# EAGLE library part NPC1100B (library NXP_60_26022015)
Low Cost Narrow Band Communication Controller The ASIC DLC-3 is a low cost narrow band communication controller MCM (Multi Carrier Modulation) and power line chip. The integrated ARMÒ CortexTM CPU, memory and common interfaces makes it possible to build different systems with a minimum of external components. For communication with DLC-3 the most popular interfaces like Ethernet MII, SPI, several freely configurable serial interfaces and general IO ports for CPU and DSC are included. The ASIC includes all components for a power-line communication while Analog Front End and Power Amplifier are already integrated. With its On-Chip Power-Factor-Correction, Ballast Control and 4 PWM outputs the LCI is a optimal solution for lighting control units. The freely configurable serial interfaces makes it easy to build electronic power meters for smart-metering applications. AAL Eindhoven MK
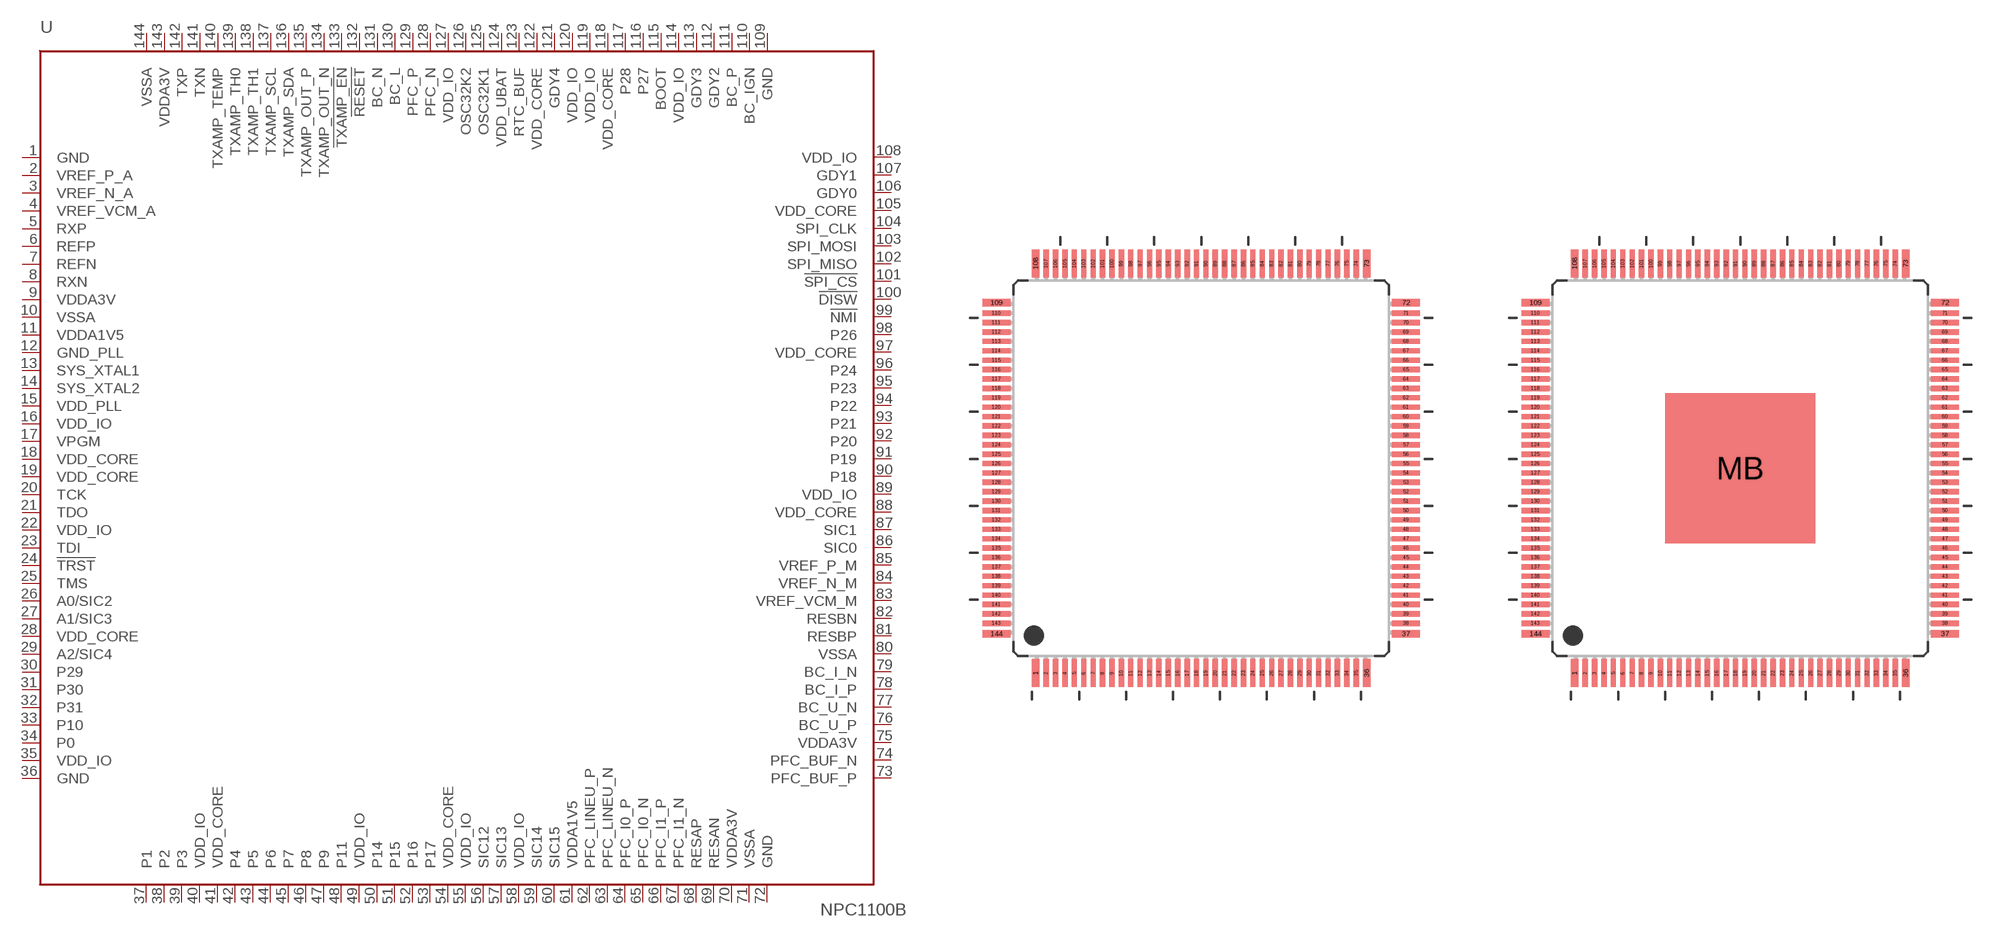
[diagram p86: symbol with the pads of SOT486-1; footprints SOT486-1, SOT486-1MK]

Designator prefix U

## NPC1100B  [SOT486-1]
1  GND
2  VREF_P_A
3  VREF_N_A
4  VREF_VCM_A
5  RXP
6  REFP
7  REFN
8  RXN
9  VDDA3V
10  VSSA
11  VDDA1V5
12  GND_PLL
13  SYS_XTAL1
14  SYS_XTAL2
15  VDD_PLL
16  VDD_IO
17  VPGM
18  VDD_CORE
19  VDD_CORE
20  TCK
21  TDO
22  VDD_IO
23  TDI
24  !TRST!
25  TMS
26  A0/SIC2
27  A1/SIC3
28  VDD_CORE
29  A2/SIC4
30  P29
31  P30
32  P31
33  P10
34  P0
35  VDD_IO
36  GND
37  P1
38  P2
39  P3
40  VDD_IO
41  VDD_CORE
42  P4
43  P5
44  P6
45  P7
46  P8
47  P9
48  P11
49  VDD_IO
50  P14
51  P15
52  P16
53  P17
54  VDD_CORE
55  VDD_IO
56  SIC12
57  SIC13
58  VDD_IO
59  SIC14
60  SIC15
61  VDDA1V5
62  PFC_LINEU_P
63  PFC_LINEU_N
64  PFC_I0_P
65  PFC_I0_N
66  PFC_I1_P
67  PFC_I1_N
68  RESAP
69  RESAN
70  VDDA3V
71  VSSA
72  GND
73  PFC_BUF_P
74  PFC_BUF_N
75  VDDA3V
76  BC_U_P
77  BC_U_N
78  BC_I_P
79  BC_I_N
80  VSSA
81  RESBP
82  RESBN
83  VREF_VCM_M
84  VREF_N_M
85  VREF_P_M
86  SIC0
87  SIC1
88  VDD_CORE
89  VDD_IO
90  P18
91  P19
92  P20
93  P21
94  P22
95  P23
96  P24
97  VDD_CORE
98  P26
99  !NMI!
100  !DISW!
101  !SPI_CS!
102  SPI_MISO
103  SPI_MOSI
104  SPI_CLK
105  VDD_CORE
106  GDY0
107  GDY1
108  VDD_IO
109  GND
110  BC_IGN
111  BC_P
112  GDY2
113  GDY3
114  VDD_IO
115  BOOT
116  P27
117  P28
118  VDD_CORE
119  VDD_IO
120  VDD_IO
121  GDY4
122  VDD_CORE
123  RTC_BUF
124  VDD_UBAT
125  OSC32K1
126  OSC32K2
127  VDD_IO
128  PFC_N
129  PFC_P
130  BC_L
131  BC_N
132  !RESET!
133  !TXAMP_EN!
134  TXAMP_OUT_N
135  TXAMP_OUT_P
136  TXAMP_SDA
137  TXAMP_SCL
138  TXAMP_TH1
139  TXAMP_TH0
140  TXAMP_TEMP
141  TXN
142  TXP
143  VDDA3V
144  VSSA

## NPC1100BCP  [SOT486-1MK]
1  GND
2  VREF_P_A
3  VREF_N_A
4  VREF_VCM_A
5  RXP
6  REFP
7  REFN
8  RXN
9  VDDA3V
10  VSSA
11  VDDA1V5
12  GND_PLL
13  SYS_XTAL1
14  SYS_XTAL2
15  VDD_PLL
16  VDD_IO
17  VPGM
18  VDD_CORE
19  VDD_CORE
20  TCK
21  TDO
22  VDD_IO
23  TDI
24  !TRST!
25  TMS
26  A0/SIC2
27  A1/SIC3
28  VDD_CORE
29  A2/SIC4
30  P29
31  P30
32  P31
33  P10
34  P0
35  VDD_IO
36  GND
37  P1
38  P2
39  P3
40  VDD_IO
41  VDD_CORE
42  P4
43  P5
44  P6
45  P7
46  P8
47  P9
48  P11
49  VDD_IO
50  P14
51  P15
52  P16
53  P17
54  VDD_CORE
55  VDD_IO
56  SIC12
57  SIC13
58  VDD_IO
59  SIC14
60  SIC15
61  VDDA1V5
62  PFC_LINEU_P
63  PFC_LINEU_N
64  PFC_I0_P
65  PFC_I0_N
66  PFC_I1_P
67  PFC_I1_N
68  RESAP
69  RESAN
70  VDDA3V
71  VSSA
72  GND
73  PFC_BUF_P
74  PFC_BUF_N
75  VDDA3V
76  BC_U_P
77  BC_U_N
78  BC_I_P
79  BC_I_N
80  VSSA
81  RESBP
82  RESBN
83  VREF_VCM_M
84  VREF_N_M
85  VREF_P_M
86  SIC0
87  SIC1
88  VDD_CORE
89  VDD_IO
90  P18
91  P19
92  P20
93  P21
94  P22
95  P23
96  P24
97  VDD_CORE
98  P26
99  !NMI!
100  !DISW!
101  !SPI_CS!
102  SPI_MISO
103  SPI_MOSI
104  SPI_CLK
105  VDD_CORE
106  GDY0
107  GDY1
108  VDD_IO
109  GND
110  BC_IGN
111  BC_P
112  GDY2
113  GDY3
114  VDD_IO
115  BOOT
116  P27
117  P28
118  VDD_CORE
119  VDD_IO
120  VDD_IO
121  GDY4
122  VDD_CORE
123  RTC_BUF
124  VDD_UBAT
125  OSC32K1
126  OSC32K2
127  VDD_IO
128  PFC_N
129  PFC_P
130  BC_L
131  BC_N
132  !RESET!
133  !TXAMP_EN!
134  TXAMP_OUT_N
135  TXAMP_OUT_P
136  TXAMP_SDA
137  TXAMP_SCL
138  TXAMP_TH1
139  TXAMP_TH0
140  TXAMP_TEMP
141  TXN
142  TXP
143  VDDA3V
144  VSSA
MB  GND

## Footprint SOT486-1 (pad centres in mm)
SOT486-1 LQFP144: plastic low profile quad flat package; 144 leads; body 20 x 20 x 1.4 mm JEDEC: MS-026 IEC: 136E23
smd 0.4 x 1.5: 1 -8.81,-10.9; 36 8.81,-10.9; 73 8.81,10.9; 108 -8.81,10.9
smd 0.28 x 1.5: 2 -8.25,-10.9; 3 -7.75,-10.9; 4 -7.25,-10.9; 5 -6.75,-10.9; 6 -6.25,-10.9; 7 -5.75,-10.9; 8 -5.25,-10.9; 9 -4.75,-10.9; 10 -4.25,-10.9; 11 -3.75,-10.9; 12 -3.25,-10.9; 13 -2.75,-10.9; 14 -2.25,-10.9; 15 -1.75,-10.9; 16 -1.25,-10.9; 17 -0.75,-10.9; 18 -0.25,-10.9; 19 0.25,-10.9; 20 0.75,-10.9; 21 1.25,-10.9; 22 1.75,-10.9; 23 2.25,-10.9; 24 2.75,-10.9; 25 3.25,-10.9; 26 3.75,-10.9; 27 4.25,-10.9; 28 4.75,-10.9; 29 5.25,-10.9; 30 5.75,-10.9; 31 6.25,-10.9; 32 6.75,-10.9; 33 7.25,-10.9; 34 7.75,-10.9; 35 8.25,-10.9; 74 8.25,10.9; 75 7.75,10.9; 76 7.25,10.9; 77 6.75,10.9; 78 6.25,10.9; 79 5.75,10.9; 80 5.25,10.9; 81 4.75,10.9; 82 4.25,10.9; 83 3.75,10.9; 84 3.25,10.9; 85 2.75,10.9; 86 2.25,10.9; 87 1.75,10.9; 88 1.25,10.9; 89 0.75,10.9; 90 0.25,10.9; 91 -0.25,10.9; 92 -0.75,10.9; 93 -1.25,10.9; 94 -1.75,10.9; 95 -2.25,10.9; 96 -2.75,10.9; 97 -3.25,10.9; 98 -3.75,10.9; 99 -4.25,10.9; 100 -4.75,10.9; 101 -5.25,10.9; 102 -5.75,10.9; 103 -6.25,10.9; 104 -6.75,10.9; 105 -7.25,10.9; 106 -7.75,10.9; 107 -8.25,10.9
smd 1.5 x 0.4: 37 10.9,-8.81; 72 10.9,8.81; 109 -10.9,8.81; 144 -10.9,-8.81
smd 1.5 x 0.28: 38 10.9,-8.25; 39 10.9,-7.75; 40 10.9,-7.25; 41 10.9,-6.75; 42 10.9,-6.25; 43 10.9,-5.75; 44 10.9,-5.25; 45 10.9,-4.75; 46 10.9,-4.25; 47 10.9,-3.75; 48 10.9,-3.25; 49 10.9,-2.75; 50 10.9,-2.25; 51 10.9,-1.75; 52 10.9,-1.25; 53 10.9,-0.75; 54 10.9,-0.25; 55 10.9,0.25; 56 10.9,0.75; 57 10.9,1.25; 58 10.9,1.75; 59 10.9,2.25; 60 10.9,2.75; 61 10.9,3.25; 62 10.9,3.75; 63 10.9,4.25; 64 10.9,4.75; 65 10.9,5.25; 66 10.9,5.75; 67 10.9,6.25; 68 10.9,6.75; 69 10.9,7.25; 70 10.9,7.75; 71 10.9,8.25; 110 -10.9,8.25; 111 -10.9,7.75; 112 -10.9,7.25; 113 -10.9,6.75; 114 -10.9,6.25; 115 -10.9,5.75; 116 -10.9,5.25; 117 -10.9,4.75; 118 -10.9,4.25; 119 -10.9,3.75; 120 -10.9,3.25; 121 -10.9,2.75; 122 -10.9,2.25; 123 -10.9,1.75; 124 -10.9,1.25; 125 -10.9,0.75; 126 -10.9,0.25; 127 -10.9,-0.25; 128 -10.9,-0.75; 129 -10.9,-1.25; 130 -10.9,-1.75; 131 -10.9,-2.25; 132 -10.9,-2.75; 133 -10.9,-3.25; 134 -10.9,-3.75; 135 -10.9,-4.25; 136 -10.9,-4.75; 137 -10.9,-5.25; 138 -10.9,-5.75; 139 -10.9,-6.25; 140 -10.9,-6.75; 141 -10.9,-7.25; 142 -10.9,-7.75; 143 -10.9,-8.25

## Footprint SOT486-1MK (pad centres in mm)
smd 0.4 x 1.5: 1 -8.81,-10.9; 36 8.81,-10.9; 73 8.81,10.9; 108 -8.81,10.9
smd 0.28 x 1.5: 2 -8.25,-10.9; 3 -7.75,-10.9; 4 -7.25,-10.9; 5 -6.75,-10.9; 6 -6.25,-10.9; 7 -5.75,-10.9; 8 -5.25,-10.9; 9 -4.75,-10.9; 10 -4.25,-10.9; 11 -3.75,-10.9; 12 -3.25,-10.9; 13 -2.75,-10.9; 14 -2.25,-10.9; 15 -1.75,-10.9; 16 -1.25,-10.9; 17 -0.75,-10.9; 18 -0.25,-10.9; 19 0.25,-10.9; 20 0.75,-10.9; 21 1.25,-10.9; 22 1.75,-10.9; 23 2.25,-10.9; 24 2.75,-10.9; 25 3.25,-10.9; 26 3.75,-10.9; 27 4.25,-10.9; 28 4.75,-10.9; 29 5.25,-10.9; 30 5.75,-10.9; 31 6.25,-10.9; 32 6.75,-10.9; 33 7.25,-10.9; 34 7.75,-10.9; 35 8.25,-10.9; 74 8.25,10.9; 75 7.75,10.9; 76 7.25,10.9; 77 6.75,10.9; 78 6.25,10.9; 79 5.75,10.9; 80 5.25,10.9; 81 4.75,10.9; 82 4.25,10.9; 83 3.75,10.9; 84 3.25,10.9; 85 2.75,10.9; 86 2.25,10.9; 87 1.75,10.9; 88 1.25,10.9; 89 0.75,10.9; 90 0.25,10.9; 91 -0.25,10.9; 92 -0.75,10.9; 93 -1.25,10.9; 94 -1.75,10.9; 95 -2.25,10.9; 96 -2.75,10.9; 97 -3.25,10.9; 98 -3.75,10.9; 99 -4.25,10.9; 100 -4.75,10.9; 101 -5.25,10.9; 102 -5.75,10.9; 103 -6.25,10.9; 104 -6.75,10.9; 105 -7.25,10.9; 106 -7.75,10.9; 107 -8.25,10.9
smd 1.5 x 0.4: 37 10.9,-8.81; 72 10.9,8.81; 109 -10.9,8.81; 144 -10.9,-8.81
smd 1.5 x 0.28: 38 10.9,-8.25; 39 10.9,-7.75; 40 10.9,-7.25; 41 10.9,-6.75; 42 10.9,-6.25; 43 10.9,-5.75; 44 10.9,-5.25; 45 10.9,-4.75; 46 10.9,-4.25; 47 10.9,-3.75; 48 10.9,-3.25; 49 10.9,-2.75; 50 10.9,-2.25; 51 10.9,-1.75; 52 10.9,-1.25; 53 10.9,-0.75; 54 10.9,-0.25; 55 10.9,0.25; 56 10.9,0.75; 57 10.9,1.25; 58 10.9,1.75; 59 10.9,2.25; 60 10.9,2.75; 61 10.9,3.25; 62 10.9,3.75; 63 10.9,4.25; 64 10.9,4.75; 65 10.9,5.25; 66 10.9,5.75; 67 10.9,6.25; 68 10.9,6.75; 69 10.9,7.25; 70 10.9,7.75; 71 10.9,8.25; 110 -10.9,8.25; 111 -10.9,7.75; 112 -10.9,7.25; 113 -10.9,6.75; 114 -10.9,6.25; 115 -10.9,5.75; 116 -10.9,5.25; 117 -10.9,4.75; 118 -10.9,4.25; 119 -10.9,3.75; 120 -10.9,3.25; 121 -10.9,2.75; 122 -10.9,2.25; 123 -10.9,1.75; 124 -10.9,1.25; 125 -10.9,0.75; 126 -10.9,0.25; 127 -10.9,-0.25; 128 -10.9,-0.75; 129 -10.9,-1.25; 130 -10.9,-1.75; 131 -10.9,-2.25; 132 -10.9,-2.75; 133 -10.9,-3.25; 134 -10.9,-3.75; 135 -10.9,-4.25; 136 -10.9,-4.75; 137 -10.9,-5.25; 138 -10.9,-5.75; 139 -10.9,-6.25; 140 -10.9,-6.75; 141 -10.9,-7.25; 142 -10.9,-7.75; 143 -10.9,-8.25
smd 8 x 8: MB 0,0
